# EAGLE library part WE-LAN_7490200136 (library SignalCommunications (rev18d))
WE-LAN LAN Transformer 10/100 Base T - Compliant with IEEE 802.3, IEEE 802.3af and IEEE 802.3at standards - SMT -- Ethernet -- Power over Ethernet -- 1 Gigabit Ethernet -- Compliant with most IC's for ethernet applications like Intel, AMD, Globespan and Realtek -- Hub, Router, Switch Details see: http://katalog.we-online.de/en/pbs/WE-LAN/7490200136 2016 (C) Würth Elektronik
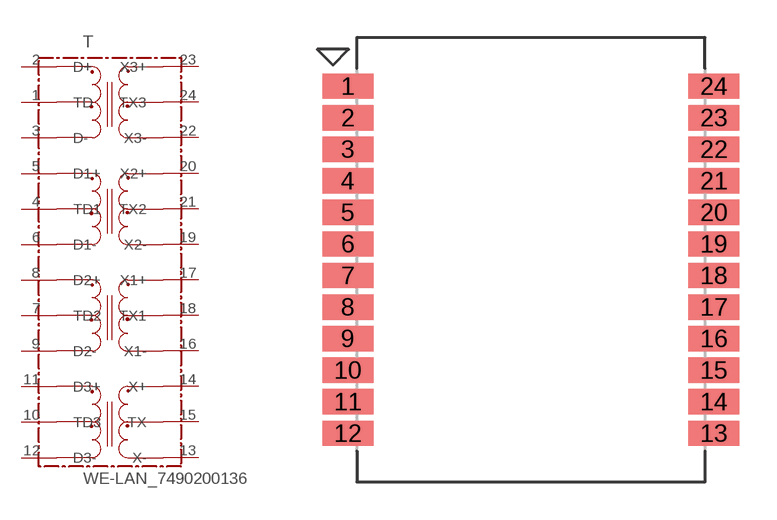
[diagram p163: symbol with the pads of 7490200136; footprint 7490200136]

Designator prefix T

## WE-LAN_7490200136  [7490200136]
1  TD
2  D+
3  D-
4  TD1
5  D1+
6  D1-
7  TD2
8  D2+
9  D2-
10  TD3
11  D3+
12  D3-
13  X-
14  X+
15  TX
16  X1-
17  X1+
18  TX1
19  X2-
20  X2+
21  TX2
22  X3-
23  X3+
24  TX3

## Footprint 7490200136 (pad centres in mm)
smd 2.05 x 1.02: 1 -7.365,6.985; 2 -7.365,5.715; 3 -7.365,4.445; 4 -7.365,3.175; 5 -7.365,1.905; 6 -7.365,0.635; 7 -7.365,-0.635; 8 -7.365,-1.905; 9 -7.365,-3.175; 10 -7.365,-4.445; 11 -7.365,-5.715; 12 -7.365,-6.985; 13 7.365,-6.985; 14 7.365,-5.715; 15 7.365,-4.445; 16 7.365,-3.175; 17 7.365,-1.905; 18 7.365,-0.635; 19 7.365,0.635; 20 7.365,1.905; 21 7.365,3.175; 22 7.365,4.445; 23 7.365,5.715; 24 7.365,6.985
